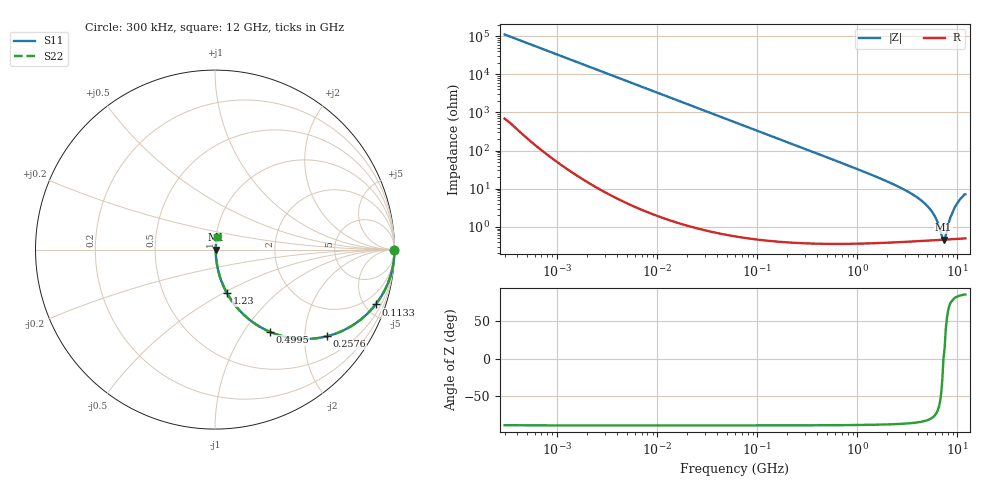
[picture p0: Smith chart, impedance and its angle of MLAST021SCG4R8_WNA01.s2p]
! MLAST021SCG4R8_WNA01  S-PARAMETER MODEL  ( General Type )
! Model Generated by TAIYO YUDEN Corporation (http://www.ty-top.com)
! Version 1.0
! TAIYO YUDEN Control No. 220901
! Copyright(c) 2022 TAIYO YUDEN CO.,LTD. All Rights Reserved.
! Product Description (link to TY-COMPAS)
! https://ds.yuden.co.jp/TYCOMPAS/or/detail?pn=MLAST021SCG4R8BWNA01&u=M
! Products Name : Multilayer Ceramic Capacitors
! Characteristics :
!  Capacitance : 4.8 pF , Rated Voltage : 25V , TCC : CG / C0G
!  Case Size : 0.25 x 0.125 / 0.0098 x 0.0049 [mm/inch] , Thickness : 0.125 / 0.0049 [mm/inch]
!  (Conditions: Temperature = 25 degC , DC Bias Current/Voltage = 0A / 0V)
! External Node Assignments :
!  1  o---| |---o  2
! GND o---------o GND
! Frequency Range : 0.3MHz  -  12000MHz  [ 401 STEP ]
# MHz S RI R 50
! Freq[MHz].  S11 Real  S11 Imag  S21 Real  S21 Imag  S12 Real  S12 Imag  S22 Real  S22 Imag
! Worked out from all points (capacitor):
!   401 points, 300 kHz to 12 GHz, reference 50 ohm
!   read as one part in series: C = 4.8 pF near 316.3 kHz
!   lowest |Z| = 458 mohm at 7.254 GHz (marker M1)
!   series resonance near 7.252 GHz, so ESL is about 100 pH
!   S11 on the Smith chart (normalised r, x): 300 kHz: open; 113.3 MHz: 1.01, -5.85; 257.6 MHz: 1.01, -2.57; 499.5 MHz: 1.01, -1.32; 1.23 GHz: 1.01, -0.52; 12 GHz: 1.01, +0.14
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0.3  1 -0.000905  6.42e-06 0.000905  6.42e-06 0.000905  1 -0.000905
1.769972  1 -0.00534  3.37e-05 0.00534  3.37e-05 0.00534  1 -0.00534
10.44266  0.999 -0.0315  0.00101 0.0315  0.00101 0.0315  0.999 -0.0315
60  0.9681 -0.1752  0.0319 0.1752  0.0319 0.1752  0.9681 -0.1752
113.3117  0.895 -0.3058  0.105 0.3058  0.105 0.3058  0.895 -0.3058
257.5933  0.6227 -0.4833  0.3773 0.4833  0.3773 0.4833  0.6227 -0.4833
353.9943  0.4663 -0.4969  0.5337 0.4969  0.5337 0.4969  0.4663 -0.4969
499.5319  0.3048 -0.4576  0.6952 0.4576  0.6952 0.4576  0.3048 -0.4576
763.2128  0.1579 -0.3605  0.8421 0.3605  0.8421 0.3605  0.1579 -0.3605
1229.528  0.0672 -0.2434  0.9328 0.2434  0.9328 0.2434  0.0672 -0.2434
2088.533  0.0243 -0.1415  0.9757 0.1415  0.9757 0.1415  0.0243 -0.1415
3454.93  0.00949 -0.0732  0.9905 0.0732  0.9905 0.0732  0.00949 -0.0732
4875.354  0.00566 -0.0369  0.9943 0.0369  0.9943 0.0369  0.00566 -0.0369
5868.704  0.00479 -0.0193  0.9952 0.0193  0.9952 0.0193  0.00479 -0.0193
6354.153  0.00461 -0.012  0.9954 0.012  0.9954 0.012  0.00461 -0.012
6879.757  0.00455 -0.00476  0.9955 0.00476  0.9955 0.00476  0.00455 -0.00476
7254.098  0.00456 2.99e-05  0.9954 -2.99e-05  0.9954 -2.99e-05  0.00456 2.99e-05
7648.807  0.00461 0.00391  0.9954 -0.00391  0.9954 -0.00391  0.00461 0.00391
8503.825  0.00496 0.0171  0.995 -0.0171  0.995 -0.0171  0.00496 0.0171
9454.42  0.00582 0.0327  0.9942 -0.0327  0.9942 -0.0327  0.00582 0.0327
11083.22  0.00829 0.0583  0.9917 -0.0583  0.9917 -0.0583  0.00829 0.0583
12000  0.00985 0.0698  0.9902 -0.0698  0.9902 -0.0698  0.00985 0.0698
